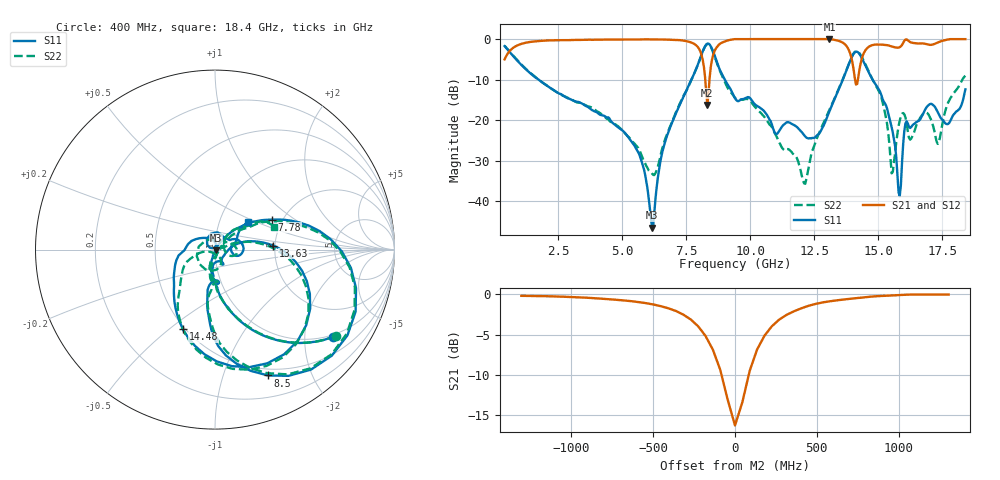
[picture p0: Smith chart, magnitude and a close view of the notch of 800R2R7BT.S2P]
!  American Technical Ceramics  Date:  10/25/10
!  One Norden Lane
!  Huntington Station,  NY.  11746-2102
!  Tel:  (631) 622-4700  Fax:  (631) 622-4748
!  Part Number  800R2R7BT.TXT  Mounting Orientation: Horizontal
!  Description: Ultra Low ESR Microwave Capacitor
!  Application: Coupling, Bypass, Tuning, DC Block, Filters, Matching
# GHZ S DB R 50
! Freq  |S11|  S11 Ph  |S21|  S21 Ph  |S12|  S12 Ph  |S22|  S22 Ph
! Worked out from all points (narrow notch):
!   401 points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, 400 MHz to 18.4 GHz, reference 50 ohm
!   highest |S21| = 0.00 dB at 13.09 GHz (marker M1); lowest = -16.3 dB at 8.32 GHz (marker M2)
!   notch at M2: 16.0 dB deep, 221 MHz wide at half that depth
!   lowest |S11| = -46.5 dB at 6.16 GHz (marker M3), VSWR 1.01, Z = 50.4 - j0.297 ohm
!   |S11| at or under -10 dB: 1.729 GHz to 7.697 GHz (5.967 GHz wide, 127 % of centre); 9.002 GHz to 13.61 GHz (4.61 GHz wide, 40.8 % of centre); 14.78 GHz to end of sweep
!   |S22| runs from -35.7 to -1.2 dB; largest |S21 - S12| = 0.0018
!   S11 on the Smith chart (normalised r, x): 400 MHz: 0.94, -2.76; 7.78 GHz: 1.77, +0.68; 8.5 GHz: 0.43, -1.42; 13.63 GHz: 1.96, +0.10; 14.48 GHz: 0.49, -0.56; 18.4 GHz: 1.38, +0.44
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0.4  -1.74 -36.4  -5.00 53.6  -5.00 53.6  -1.65 -35.6
1.345  -8.11 -72.8  -0.76 17.3  -0.76 17.3  -7.99 -72.2
3.415  -15.86 -94.0  -0.19 -5.9  -0.18 -6.0  -15.86 -94.3
5.485  -26.40 -107.1  -0.11 -20.4  -0.11 -20.4  -25.86 -92.0
6.16  -46.49 -38.5  -0.09 -25.4  -0.09 -25.4  -33.16 -36.2
6.43  -32.29 54.8  -0.09 -27.6  -0.09 -27.6  -30.38 20.0
7.78  -8.87 27.7  -1.09 -50.1  -1.10 -50.1  -8.85 25.9
8.32  -1.12 -32.9  -16.26 -31.1  -16.26 -31.1  -1.20 -32.4
8.5  -2.38 -67.2  -5.12 13.6  -5.12 13.5  -2.54 -67.2
9.4  -14.60 -96.6  -0.01 -20.4  -0.01 -20.5  -14.50 -92.1
12.1  -23.63 -55.1  -0.01 -50.3  -0.01 -50.4  -35.58 -41.9
12.415  -24.37 -30.3  -0.01 -53.2  -0.01 -53.2  -27.65 13.0
13.09  -17.79 14.7  0.00 -62.3  -0.01 -62.3  -17.42 16.8
13.63  -9.72 3.9  -0.96 -76.1  -0.96 -76.2  -9.60 0.8
14.035  -3.61 -39.6  -7.59 -91.0  -7.59 -91.0  -3.52 -41.6
14.485  -6.40 -111.9  -2.85 -31.2  -2.85 -31.2  -6.08 -109.7
15.43  -19.37 144.1  -1.63 -52.8  -1.64 -52.8  -25.95 -168.1
15.565  -23.08 117.3  -1.89 -52.6  -1.88 -52.6  -32.75 -97.5
15.835  -38.72 124.2  -1.99 -47.1  -1.99 -47.1  -20.11 -74.0
16.105  -20.27 82.2  -0.08 -52.6  -0.08 -52.6  -20.72 169.5
17.32  -18.01 -16.2  -0.84 -55.3  -0.84 -55.4  -25.84 9.7
18.4  -12.39 39.1  -0.01 -75.4  -0.01 -75.5  -9.06 21.3
